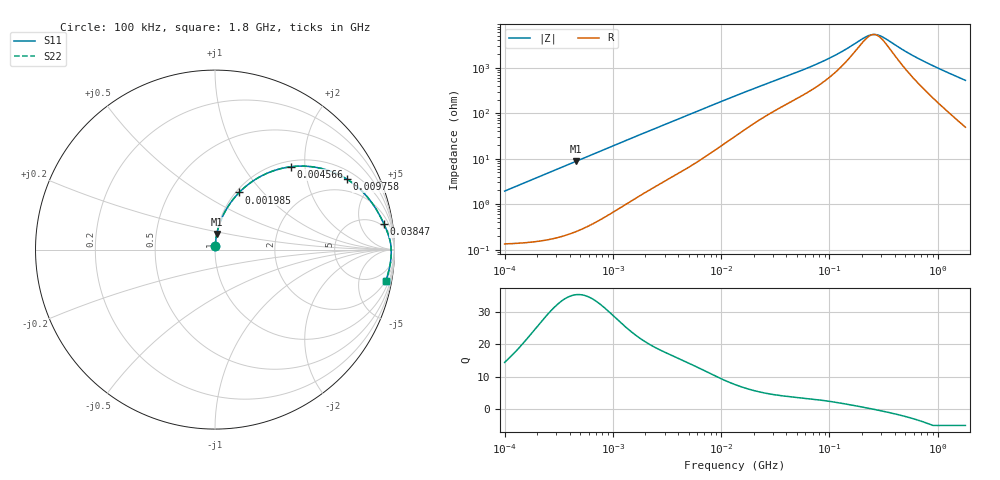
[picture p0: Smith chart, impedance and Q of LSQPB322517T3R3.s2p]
! LSQPB322517T3R3  S-PARAMETER MODEL  ( General Type )
! Model Generated by TAIYO YUDEN Corporation (http://www.ty-top.com)
! Version 2.0
! TAIYO YUDEN Control No. 100810NG22EB-FKC
! Copyright(c) 2009 TAIYO YUDEN CO.,LTD. All Rights Reserved.
! Product Description (link to TY-COMPAS)
! https://ds.yuden.co.jp/TYCOMPAS/or/detail?pn=LSQPB322517T3R3M&u=M
! Products Name : Inductors
! Characteristics :
!  Inductance : 3.3 uH , SRF(min) : 140 MHz , DC Resistance(max) : 0.144 Ohm
!  Rated Current : Saturation :1450 mA , Temp Rise : 1200 mA (40 degC)
!  Case Size : 3.2 x 2.5 / 0.126 x 0.098 [mm/inch] , Thickness : 1.7 / 0.068 [mm/inch]
!  (Conditions: Temperature = 25 degC , DC Bias Current/Voltage = 0A / 0V)
! External Node Assignments :
!  1  o---GGG---o  2
! GND o---------o GND
! Frequency Range : 0.1MHz  -  1800MHz  [ 402 STEP ]
# MHz S RI R 50
! Freq[MHz].  S11 Real  S11 Imag  S21 Real  S21 Imag  S12 Real  S12 Imag  S22 Real  S22 Imag
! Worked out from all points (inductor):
!   401 points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, 100 kHz to 1.8 GHz, reference 50 ohm
!   read as one part in series: L = 3.07 uH near 105 kHz
!   highest Q = 35.4 at 456.6 kHz (marker M1), where L = 3.07 uH
!   self-resonance near 255.4 MHz
!   S11 on the Smith chart (normalised r, x): 100 kHz: 1.00, +0.04; 1.985 MHz: 1.04, +0.75; 4.566 MHz: 1.11, +1.68; 9.758 MHz: 1.37, +3.51; 38.47 MHz: 4, +12; 1.8 GHz: 2, -11
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0.1  0.0017 0.0192  0.9983 -0.0192  0.9983 -0.0192  0.0017 0.0192
0.456633  0.0101 0.0868  0.9899 -0.0868  0.9899 -0.0868  0.0101 0.0868
0.516129  0.0125 0.0978  0.9875 -0.0978  0.9875 -0.0978  0.0125 0.0978
1.130264  0.0514 0.2033  0.9486 -0.2033  0.9486 -0.2033  0.0514 0.2033
1.985446  0.1349 0.3185  0.8651 -0.3185  0.8651 -0.3185  0.1349 0.3185
2.66389  0.212 0.3826  0.788 -0.3826  0.788 -0.3826  0.212 0.3826
4.566214  0.421 0.4613  0.579 -0.4613  0.579 -0.4613  0.421 0.4613
6.434145  0.5756 0.4559  0.4244 -0.4559  0.4244 -0.4559  0.5756 0.4559
9.75753  0.7362 0.3916  0.2638 -0.3916  0.2638 -0.3916  0.7362 0.3916
13.41641  0.8218 0.3227  0.1782 -0.3227  0.1782 -0.3227  0.8218 0.3227
20.85084  0.8932 0.2325  0.1068 -0.2325  0.1068 -0.2325  0.8932 0.2325
38.46609  0.9421 0.141  0.0579 -0.141  0.0579 -0.141  0.9421 0.141
69.24595  0.9659 0.0822  0.0341 -0.0822  0.0341 -0.0822  0.9659 0.0822
115.8234  0.9764 0.0444  0.0236 -0.0444  0.0236 -0.0444  0.9764 0.0444
208.5031  0.9812 0.0106  0.0188 -0.0106  0.0188 -0.0106  0.9812 0.0106
235.6695  0.9816 0.0042  0.0184 -0.0042  0.0184 -0.0042  0.9816 0.0042
279.7504  0.9819 -0.00477  0.0181 0.00477  0.0181 0.00477  0.9819 -0.00477
357.3983  0.9819 -0.018  0.0181 0.018  0.0181 0.018  0.9819 -0.018
503.6016  0.981 -0.0384  0.019 0.0384  0.019 0.0384  0.981 -0.0384
709.6131  0.9785 -0.0634  0.0215 0.0634  0.0215 0.0634  0.9785 -0.0634
1158.204  0.9697 -0.1121  0.0303 0.1121  0.0303 0.1121  0.9697 -0.1121
1800  0.9501 -0.1759  0.0499 0.1759  0.0499 0.1759  0.9501 -0.1759
